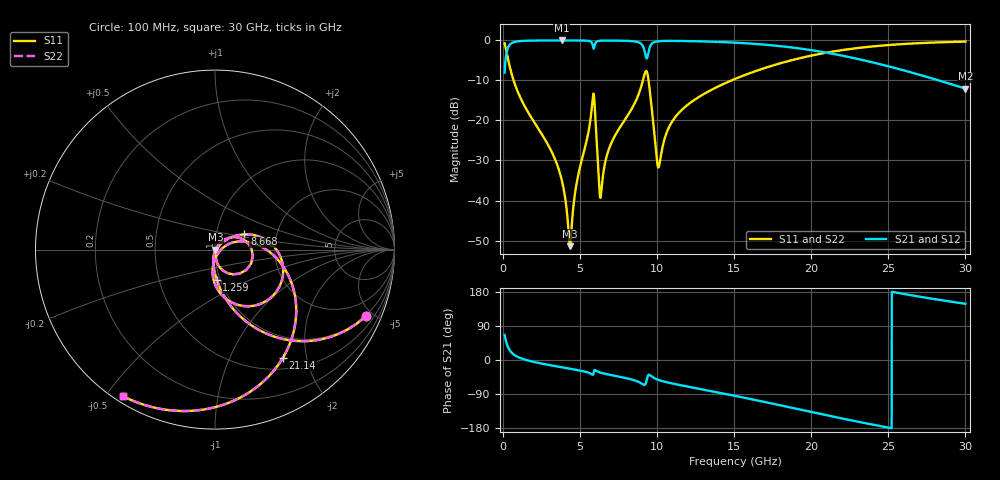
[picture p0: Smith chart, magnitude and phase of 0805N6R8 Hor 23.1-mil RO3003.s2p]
# GHz S MA R 50
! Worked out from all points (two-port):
!   3201 points, 100 MHz to 30 GHz, reference 50 ohm
!   highest |S21| = -0.02 dB at 3.819 GHz (marker M1); lowest = -12.1 dB at 30 GHz (marker M2)
!   |S21| within 3 dB of the highest: 231.1 MHz to 9.207 GHz (8.976 GHz wide, 190 % of centre); 9.432 GHz to 20.91 GHz (11.48 GHz wide, 75.7 % of centre)
!   lowest |S11| = -51.4 dB at 4.342 GHz (marker M3), VSWR 1.01, Z = 50.2 - j0.102 ohm
!   |S11| at or under -10 dB: 683.1 MHz to 9.074 GHz (8.39 GHz wide, 172 % of centre); 9.439 GHz to 14.83 GHz (5.386 GHz wide, 44.4 % of centre)
!   |S22| runs from -51.4 to -0.3 dB; largest |S21 - S12| = 0
!   S11 on the Smith chart (normalised r, x): 100 MHz: 0.96, -4.54; 1.259 GHz: 0.96, -0.34; 8.668 GHz: 1.37, +0.24; 21.14 GHz: 0.66, -1.61; 30 GHz: 0.02, -0.55
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0.1  0.9182 -23.8  0.3958 66.1  0.3958 66.1  0.9182 -23.8
0.511125  0.4097 -68.4  0.9115 21.5  0.9115 21.5  0.4097 -68.4
1.258625  0.1702 -86.5  0.9841 3.1  0.9841 3.1  0.1702 -86.5
3.818812  0.01764 -101.7  0.9974 -19.3  0.9974 -19.3  0.01764 -101.7
4.342062  0.00269 -22.2  0.9972 -23.0  0.9972 -23.0  0.00269 -22.2
5.089563  0.03106 53.6  0.9952 -28.7  0.9952 -28.7  0.03106 53.6
5.85575  0.2136 -9.4  0.8048 -36.4  0.8048 -36.4  0.2136 -9.4
5.986562  0.1098 -73.2  0.9206 -27.0  0.9206 -27.0  0.1098 -73.2
6.2295  0.0164 -65.0  0.9859 -32.3  0.9859 -32.3  0.0164 -65.0
6.360313  0.01219 6.4  0.9904 -33.9  0.9904 -33.9  0.01219 6.4
6.958312  0.04875 44.3  0.9931 -39.3  0.9931 -39.3  0.04875 44.3
8.668219  0.1846 27.3  0.9602 -55.7  0.9602 -55.7  0.1846 27.3
9.032625  0.2955 9.7  0.8725 -63.3  0.8725 -63.3  0.2955 9.7
9.340969  0.4006 -47.4  0.5992 -49.1  0.5992 -49.1  0.4006 -47.4
9.602594  0.17 -92.6  0.8826 -42.2  0.8826 -42.2  0.17 -92.6
10.06978  0.02587 -39.3  0.9744 -52.3  0.9744 -52.3  0.02587 -39.3
11.40594  0.1243 20.5  0.9834 -65.6  0.9834 -65.6  0.1243 20.5
15.05  0.3298 -5.9  0.9363 -94.6  0.9363 -94.6  0.3298 -5.9
20.03956  0.6473 -48.2  0.7526 -137.5  0.7526 -137.5  0.6473 -48.2
21.14213  0.7108 -57.8  0.6934 -147.0  0.6934 -147.0  0.7108 -57.8
25.01978  0.8747 -89.1  0.4735 -178.5  0.4735 -178.5  0.8747 -89.1
30  0.9648 -122.3  0.2496 148.3  0.2496 148.3  0.9648 -122.3
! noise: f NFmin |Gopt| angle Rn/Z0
0.1  0.0007661  0.9197  1.005  0.002108
3.417  0.006492  0.7107  18.27  0.004312
6.743  0.01489  0.7497  35.33  0.0109
10.06  0.03781  0.8484  51.94  0.04295
13.39  0.02289  0.7017  66.86  0.01061
16.7  0.02773  0.7017  80.95  0.01077
20.03  0.03507  0.7229  94.39  0.01194
23.35  0.04533  0.755  107.3  0.01361
26.67  0.06031  0.795  120  0.01577
30  0.08355  0.8395  132.8  0.01837
